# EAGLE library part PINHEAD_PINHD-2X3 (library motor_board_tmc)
PIN HEADER
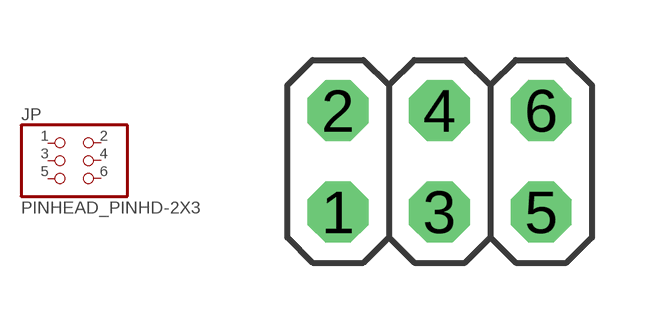
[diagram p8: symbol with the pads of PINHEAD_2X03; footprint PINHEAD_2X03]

Designator prefix JP

## PINHEAD_PINHD-2X3  [PINHEAD_2X03]
1  1  pas
2  2  pas
3  3  pas
4  4  pas
5  5  pas
6  6  pas

## Footprint PINHEAD_2X03 (pad centres in mm)
PIN HEADER
drill 1.016 octagon: 1 -2.54,-1.27; 2 -2.54,1.27; 3 0,-1.27; 4 0,1.27; 5 2.54,-1.27; 6 2.54,1.27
